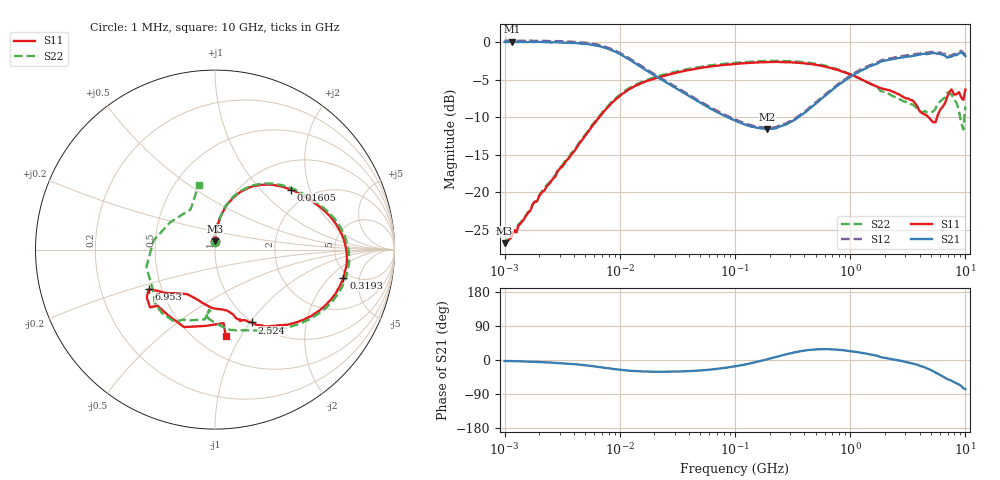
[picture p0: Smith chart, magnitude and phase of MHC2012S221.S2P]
!Agilent Technologies,E5071C,MY46111244,A.11.31
!Date: Fri May 17 14:37:17 2019
!Data & Calibration Information:
!Freq	S11:SOLT2(ON)	S21:SOLT2(ON)	S12:SOLT2(ON)	S22:SOLT2(ON)
# Hz S dB R 50
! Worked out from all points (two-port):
!   201 points, 1 MHz to 10 GHz, reference 50 ohm
!   highest |S21| = 0.07 dB at 1.159 MHz (marker M1); lowest = -11.6 dB at 190.5 MHz (marker M2)
!   |S21| within 3 dB of the highest: start of sweep to 13.98 MHz; 1.667 GHz to end of sweep
!   lowest |S11| = -26.7 dB at 1 MHz (marker M3), VSWR 1.10, Z = 49.8 + j4.59 ohm
!   |S11| at or under -10 dB: start of sweep to 6.64 MHz; 4.788 GHz to 5.682 GHz (894.4 MHz wide, 17.1 % of centre)
!   |S22| runs from -27.1 to -2.5 dB; largest |S21 - S12| = 0.026
!   S11 on the Smith chart (normalised r, x): 1 MHz: 1.00, +0.09; 16.05 MHz: 1.60, +1.51; 319.3 MHz: 4.41, -2.97; 2.524 GHz: 1.00, -1.02; 6.953 GHz: 0.42, -0.23; 10 GHz: 0.69, -0.86
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1000000  -26.75 90.0  0.03 -2.5  0.17 -2.5  -27.15 90.7
1159128  -25.80 93.9  0.07 -3.0  0.19 -2.9  -25.64 95.2
4810209  -12.82 77.0  -0.23 -13.3  -0.05 -13.3  -12.69 77.4
9165665  -7.66 58.6  -1.29 -24.3  -1.14 -24.4  -7.50 58.6
1.605417e7  -5.35 38.2  -3.52 -30.3  -3.36 -30.4  -5.20 38.1
2.206931e7  -4.66 29.8  -4.83 -30.9  -4.67 -31.0  -4.50 29.7
1.047129e8  -2.87 4.9  -10.58 -15.7  -10.41 -15.7  -2.73 4.9
1.905461e8  -2.66 -3.2  -11.55 1.8  -11.39 1.8  -2.51 -3.4
3.192505e8  -2.70 -12.3  -10.47 19.3  -10.31 19.3  -2.55 -12.4
4.810209e8  -2.99 -21.4  -8.44 27.5  -8.28 27.5  -2.85 -21.8
1.047129e9  -4.43 -42.9  -4.45 22.8  -4.28 22.8  -4.40 -45.3
2.206931e9  -6.41 -61.3  -2.33 3.3  -2.16 3.3  -6.95 -80.8
2.524434e9  -6.82 -62.9  -2.18 -0.2  -1.99 -0.2  -7.49 -86.5
3.801894e9  -8.48 -74.2  -1.72 -12.3  -1.55 -12.4  -8.86 -97.0
5.495409e9  -10.67 -122.0  -1.49 -33.0  -1.32 -33.0  -8.89 -96.6
6.952868e9  -7.32 -149.1  -2.07 -50.1  -1.87 -50.2  -6.71 -119.3
7.585776e9  -6.30 -138.4  -1.93 -54.7  -1.77 -54.6  -6.97 -138.5
7.988146e9  -6.98 -135.7  -1.76 -58.6  -1.59 -58.5  -7.69 -146.8
8.390517e9  -6.94 -125.0  -1.74 -61.6  -1.58 -61.6  -8.08 -165.8
8.792888e9  -6.65 -111.8  -1.49 -64.5  -1.29 -64.7  -9.21 171.5
9.597629e9  -7.69 -83.4  -1.59 -74.4  -1.42 -74.4  -11.62 121.1
1e10  -6.32 -82.9  -1.86 -77.1  -1.68 -77.0  -8.55 104.0
